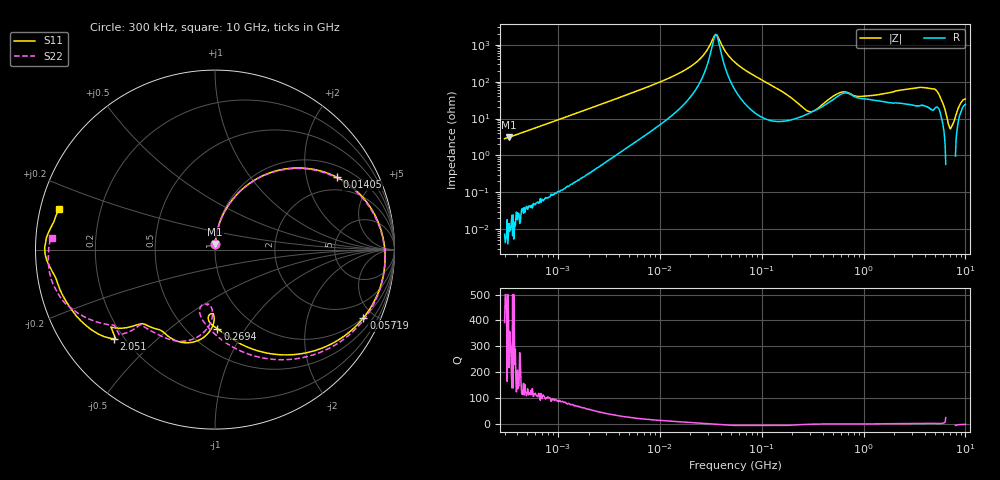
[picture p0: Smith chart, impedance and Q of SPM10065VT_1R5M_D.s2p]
! S-Parameter Data Generated by TDK Corporation
! Copyright(C) 2020 TDK Corporation.
! All Rights Reserved.
! TDK P/N: SPM10065VT-1R5M-D (Inductor)
! Property: L=1.5uH at 100kHz
! Size(LxWxT): 10.5x10x6.5mm
! Model Type: s2p (Touchstone File Format Version 1.0)
! Frequency: DC=Yes Start=0.3MHz Stop=10000MHz 802points Log-sweep
! Model Generated on Apr. 23, 2020
! Port Assignments:
!  1 ---@@@--- 2
! Applicable Conditions:
!  Temperature = 25 degC
!  DC Bias Current = 0 A
!  Small Signal Operation
! Terms and conditions regarding TDK Simulation Models
! (1)This simulation model is being provided solely for informational purposes. Please refer to the specifications of the products in terms of detailed characteristics of such products.
! (2)In no event shall TDK Corporation of any of its subsidiaries be liable for any loss or damage arising, directly or indirectly,
!  From any information contained in this simulation model, including, but not limited to loss or damages arising from any inaccuracies, omissions or errors in connection with such information.
! (3)Any and all copyrights on this simulation model are owned by TDK Corporation.
!  Duplication or redistribution of this simulation model without prior written permission from TDK Corporation is prohibited.
! (4)This simulation model is subject to any modification or change without any prior notice.
! (5)Neither TDK Corporation nor any of its subsidiaries shall make any warranty, express or implied,
!  Including but not limited to the correctness, implied warranties of merchantability and fitness for a particular purpose with respect to this simulation models.
! (6)The use of this simulation model shall be deemed to have consented to the terms and conditions hereof.
# Hz S MA R 50
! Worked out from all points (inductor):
!   801 points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, 300 kHz to 10 GHz, reference 50 ohm
!   read as one part in series: L = 1.49 uH near 318.3 kHz
!   highest Q = 437 at 332.1 kHz (marker M1), where L = 1.5 uH
!   self-resonance near 35.56 MHz
!   S11 on the Smith chart (normalised r, x): 300 kHz: 1.00, +0.06; 14.05 MHz: 1.42, +3.05; 57.19 MHz: 0.98, -4.35; 269.4 MHz: 0.69, -0.75; 2.051 GHz: 0.16, -0.37; 10 GHz: 0.05, +0.13
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300000  0.029 89.5  0.9989 -1.6  0.9991 -1.6  0.02906 89.1
332090  0.03173 88.9  0.9986 -1.7  0.9991 -1.8  0.03179 88.8
1713600  0.153 80.1  0.986 -9.0  0.9856 -9.1  0.153 80.0
4425256  0.3698 65.7  0.9163 -22.4  0.9162 -22.4  0.3699 65.5
9671944  0.6577 43.8  0.7101 -42.5  0.7099 -42.5  0.6578 43.4
1.405002e7  0.7908 30.6  0.5404 -54.1  0.5403 -54.1  0.7909 30.1
2.441527e7  0.9211 9.8  0.2338 -67.8  0.2337 -67.8  0.9214 8.9
3.555278e7  0.9498 -4.9  0.04972 -5.6  0.04972 -5.6  0.9499 -6.2
4.564296e7  0.9397 -15.1  0.1605 56.7  0.1605 56.7  0.9399 -16.8
5.477226e7  0.9172 -22.9  0.2679 56.0  0.2678 56.0  0.9173 -24.9
5.718581e7  0.91 -24.8  0.2933 55.1  0.2932 55.1  0.91 -26.9
1.145169e8  0.7085 -55.9  0.6465 27.0  0.6463 27.0  0.7066 -60.2
1.810762e8  0.5442 -74.8  0.7703 4.2  0.77 4.2  0.5356 -81.7
2.694285e8  0.4412 -88.3  0.7851 -17.2  0.7848 -17.2  0.4099 -98.5
3.126428e8  0.4077 -94.0  0.7555 -25.1  0.7552 -25.1  0.3526 -104.1
5.105874e8  0.418 -91.3  0.6338 -55.7  0.6336 -55.6  0.3355 -92.7
7.497801e8  0.552 -115.3  0.4543 -65.3  0.4541 -65.3  0.5314 -107.1
1.133369e9  0.5637 -130.6  0.4148 -93.7  0.4146 -93.7  0.5791 -129.7
1.767019e9  0.6643 -139.0  0.2629 -141.7  0.2627 -141.6  0.6557 -136.1
2.051294e9  0.7504 -138.5  0.1918 -157.8  0.1917 -157.7  0.7081 -143.6
5.099159e9  0.9022 -170.0  0.0206 171.1  0.02055 171.1  0.9115 -165.2
1e10  0.8978 165.5  0.02199 137.8  0.02192 138.2  0.909 176.0
